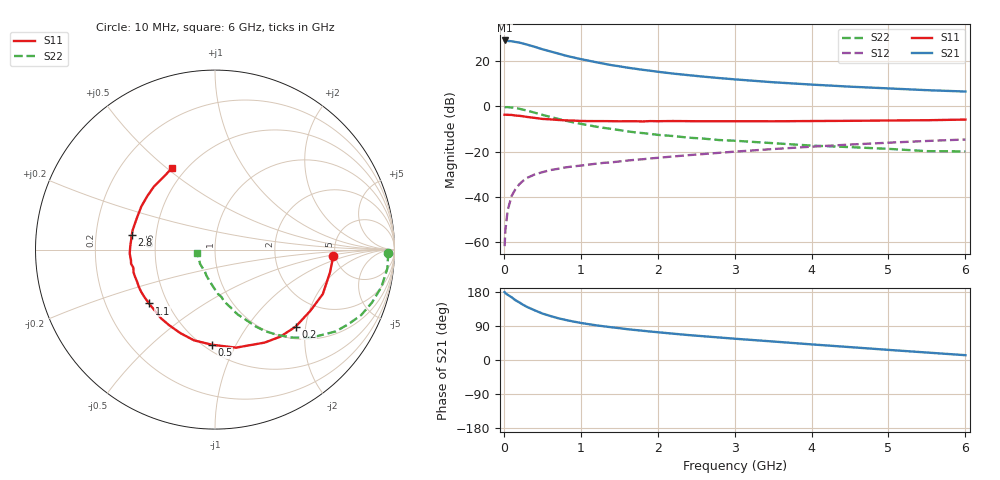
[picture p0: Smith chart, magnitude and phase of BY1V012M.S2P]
! SIEMENS Small Signal Semiconductors
! BFY420
! Si NPN RF SIEGET Grounded Emitter Transistor in MICRO-X
! VCE = 1 V  IC = 12 mA
! Common Emitter S-Parameters:  October  1996
# GHz  S  MA  R  50
!  f  S11  S21  S12  S22
! GHz  MAG  ANG  MAG  ANG  MAG  ANG  MAG  ANG
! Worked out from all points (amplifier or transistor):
!   36 points, 10 MHz to 6 GHz, reference 50 ohm
!   highest |S21| = 29.3 dB at 10 MHz (marker M1)
!   |S21| within 3 dB of that: start of sweep to 418.3 MHz
!   unconditionally stable (mu >= 1): 2.246 GHz to end of sweep
!   at 250 MHz: K = 0.22, MSG = 30.4 dB, |S12| = -33.0 dB
!   at 1.4 GHz: K = 0.82, MSG = 21.5 dB, |S12| = -24.8 dB
!   at 6 GHz: K = 1.11, MAG = 8.6 dB, |S12| = -14.6 dB
!   S11 on the Smith chart (normalised r, x): 10 MHz: 4.74, -0.55; 200 MHz: 1.26, -1.76; 500 MHz: 0.55, -0.81; 1.1 GHz: 0.40, -0.31; 2.8 GHz: 0.36, +0.07; 6 GHz: 0.42, +0.52
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0.01  0.6557 -2.9  29.09 179.2  0.0008 88.2  0.9648 -1.0
0.02  0.6577 -4.8  28.98 176.5  0.0018 90.0  0.9649 -2.2
0.05  0.6532 -11.2  28.33 172.1  0.005 85.2  0.9662 -6.2
0.1  0.6497 -22.4  27.96 165.7  0.0103 79.3  0.9505 -12.6
0.15  0.6312 -32.8  26.96 157.9  0.0146 75.0  0.9227 -18.7
0.2  0.6214 -43.7  26.11 152.1  0.0188 71.4  0.892 -24.2
0.25  0.6065 -53.1  24.86 145.7  0.0225 67.2  0.8498 -29.4
0.3  0.5873 -61.9  23.6 140.2  0.026 64.1  0.8128 -34.1
0.4  0.5587 -77.9  21.07 131.2  0.0311 58.7  0.7293 -42.2
0.5  0.5304 -91.8  18.6 122.7  0.0349 55.0  0.6535 -48.6
0.6  0.5188 -103.1  16.7 116.4  0.0388 52.2  0.5891 -53.8
0.7  0.5038 -112.5  15.02 110.6  0.0414 50.7  0.5346 -58.3
0.8  0.4927 -121.2  13.47 105.8  0.0446 48.6  0.4859 -62.0
0.9  0.4869 -128.1  12.26 101.6  0.0469 47.9  0.4452 -64.8
1.1  0.4744 -140.8  10.39 94.6  0.0514 47.8  0.3839 -70.6
1.6  0.4706 -161.4  7.282 81.4  0.063 46.8  0.2825 -80.8
2.2  0.4757 -177.3  5.362 69.5  0.0779 46.0  0.2212 -90.2
2.8  0.471 170.3  4.268 59.4  0.0939 44.2  0.1803 -98.8
3.5  0.4696 157.9  3.446 48.8  0.1138 40.5  0.1537 -107.9
4.5  0.4808 141.7  2.751 34.0  0.1431 33.2  0.1256 -122.3
5.5  0.4956 125.4  2.299 19.7  0.172 24.3  0.1023 -150.5
6  0.5131 118.0  2.145 12.7  0.1855 19.6  0.1011 -168.3
